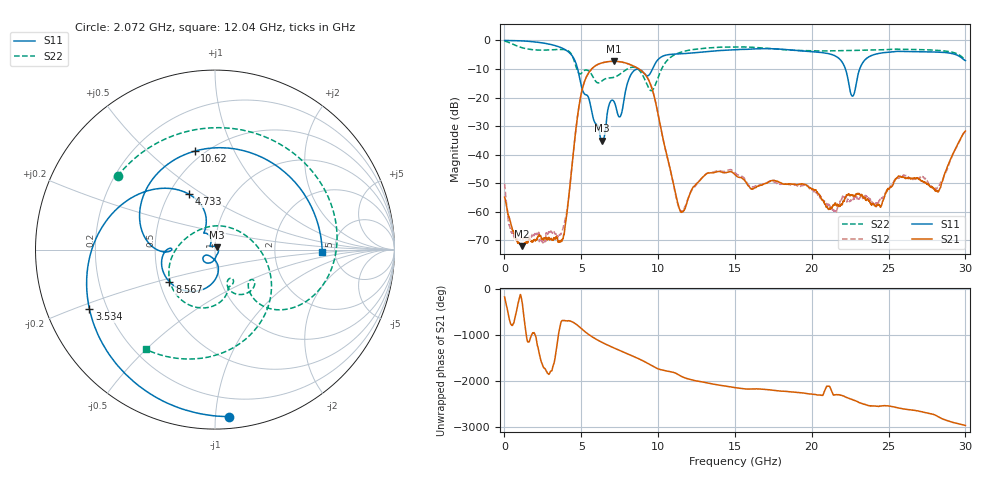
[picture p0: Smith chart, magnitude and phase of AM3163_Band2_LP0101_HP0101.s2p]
!Agilent Technologies,E8364B,MY43040894,A.07.50.67
!Agilent E8364B: A.07.50.67
!Date: Thursday, August 20, 2020 11:12:39
!Correction: S11(Full 2 Port(1,2))
!S21(Full 2 Port(1,2))
!S12(Full 2 Port(1,2))
!S22(Full 2 Port(1,2))
!S2P File: Measurements: S11, S21, S12, S22:
# Hz S  dB  R 50
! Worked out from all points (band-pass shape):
!   3201 points, 10 MHz to 30 GHz, reference 50 ohm
!   highest |S21| = -7.30 dB at 7.142 GHz (marker M1); lowest = -72.0 dB at 1.153 GHz (marker M2)
!   |S21| within 3 dB of the highest: 5.627 GHz to 8.835 GHz (3.208 GHz wide, 44.4 % of centre)
!   lowest |S11| = -35.1 dB at 6.364 GHz (marker M3), VSWR 1.04, Z = 51.1 + j1.38 ohm
!   |S11| at or under -10 dB: 4.765 GHz to 9.635 GHz (4.87 GHz wide, 67.6 % of centre); 22.19 GHz to 23.12 GHz (928.4 MHz wide, 4.1 % of centre)
!   |S22| runs from -17.6 to -0.2 dB; largest |S21 - S12| = 0.0046
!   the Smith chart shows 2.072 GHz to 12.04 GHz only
!   S11 on the Smith chart (normalised r, x): 2.072 GHz: 0.07, -1.08; 3.534 GHz: 0.13, -0.22; 4.733 GHz: 0.63, +0.44; 8.567 GHz: 0.56, -0.22; 10.62 GHz: 0.45, +0.71; 12.04 GHz: 3.96, -0.18
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1e7  -0.02 -2.8  -54.88 -164.4  -50.15 -26.7  -0.24 -10.2
5.535688e8  -0.07 -22.3  -66.68 -41.4  -68.06 118.5  -1.39 -77.7
1.153369e9  -0.18 -46.8  -72.03 76.2  -69.59 112.9  -2.58 -142.3
2.071812e9  -0.59 -85.4  -69.93 5.5  -67.95 -174.4  -3.35 143.0
3.533825e9  -2.22 -154.5  -70.57 138.8  -68.52 -82.7  -3.16 41.2
3.955559e9  -3.25 -179.7  -64.62 40.2  -62.57 74.7  -3.28 7.8
4.733425e9  -9.35 115.1  -27.48 -54.0  -27.50 -54.5  -10.50 -50.3
5.014581e9  -16.21 108.5  -18.24 -134.6  -18.26 -134.9  -11.46 -38.7
6.364131e9  -35.12 50.2  -7.84 -74.2  -7.86 -74.3  -14.10 -58.9
7.141997e9  -21.51 -143.4  -7.30 164.6  -7.31 164.4  -12.90 -70.7
8.566522e9  -10.15 -144.8  -9.43 -41.9  -9.43 -41.8  -9.60 -130.3
1.000979e10  -6.64 154.5  -26.21 70.9  -26.11 70.0  -12.79 6.6
1.061896e10  -5.03 101.5  -41.27 24.9  -41.36 22.4  -6.84 -52.2
1.145306e10  -4.68 37.9  -59.85 -79.1  -59.69 -81.2  -4.19 -99.9
1.204349e10  -4.47 -1.4  -54.04 -154.6  -54.05 -153.9  -3.40 -124.8
1.5005e10  -3.21 -142.7  -47.02 23.3  -46.27 24.4  -2.26 132.8
1.771347e10  -2.98 94.6  -49.29 -42.0  -50.03 -45.3  -3.04 30.9
2.000958e10  -3.95 -27.5  -52.06 -119.3  -52.24 -116.2  -3.67 -50.2
2.265245e10  -19.51 -107.3  -54.27 123.0  -56.21 61.9  -3.53 -124.8
2.500479e10  -4.13 -150.8  -51.97 -16.2  -52.22 -22.4  -3.20 177.7
2.824746e10  -4.11 107.4  -52.87 108.5  -51.29 103.4  -3.50 91.3
3e10  -7.08 41.7  -31.75 -78.3  -31.84 -78.8  -6.69 37.4
